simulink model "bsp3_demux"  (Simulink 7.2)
settings: Solver=VariableStepDiscrete  SolverMode=SingleTasking  StartTime=0.0  StopTime=10.0  FixedStep=0.01  RelTol=1e-3

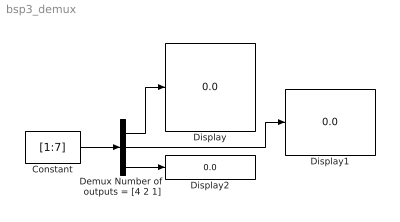
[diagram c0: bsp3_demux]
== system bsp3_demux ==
  Constant : Constant  Value=[1:7]  OutDataType=sfix(16)  OutScaling=2^0
  Demux Number of  outputs = [4 2 1] : Demux  Outputs=[4 2 1]
  Display : Display
  Display1 : Display
  Display2 : Display
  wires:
  Constant/1 -> Demux Number of  outputs = [4 2 1]/1
  Demux Number of  outputs = [4 2 1]/1 -> Display/1
  Demux Number of  outputs = [4 2 1]/2 -> Display1/1
  Demux Number of  outputs = [4 2 1]/3 -> Display2/1
